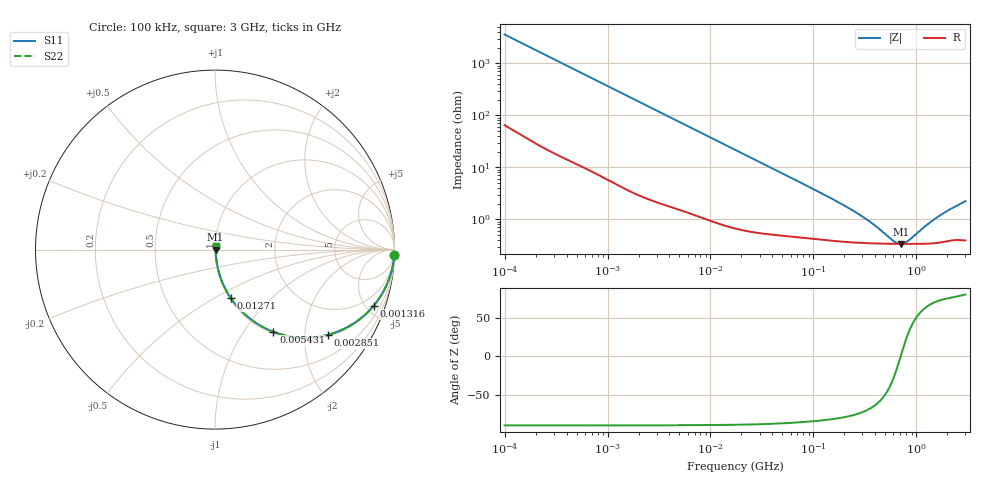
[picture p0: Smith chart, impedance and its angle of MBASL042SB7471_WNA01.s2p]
! MBASL042SB7471_WNA01  S-PARAMETER MODEL  ( Standard Model )
! Model Generated by TAIYO YUDEN Corporation (https://www.yuden.co.jp/en/)
! Version 1.0
! TAIYO YUDEN Control No. 250312
! Copyright(c) 2025 TAIYO YUDEN CO.,LTD. All Rights Reserved.
! Product Description (link to TY-COMPAS)
! https://ds.yuden.co.jp/TYCOMPAS/or/detail?pn=MBASL042SB7471KWNA01&u=M
! Products Name : Multilayer Ceramic Capacitors
! Characteristics :
!  Capacitance : 470 [pF] , Rated Voltage : 10 [V] , TCC : X7R
!  Case Size : 0.4 x 0.2 / 0.016 x 0.008 [mm/inch] , Thickness : 0.2 / 0.008 [mm/inch]
!  (Conditions: Temperature = 25 [degC] , DC Bias Voltage = 0 [V])
! External Node Assignments :
!  1  o---| |---o  2
! GND o---------o GND
! Frequency Range : 100kHz  -  3GHz  [ 401 STEP ]
# MHZ S RI R 50
! Freq[MHz].  S11 Real  S11 Imag  S21 Real  S21 Imag  S12 Real  S12 Imag  S22 Real  S22 Imag
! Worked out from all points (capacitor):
!   401 points, 100 kHz to 3 GHz, reference 50 ohm
!   read as one part in series: C = 440 pF near 105.3 kHz
!   lowest |Z| = 337 mohm at 708.5 MHz (marker M1)
!   series resonance near 704.3 MHz, so ESL is about 120 pH
!   S11 on the Smith chart (normalised r, x): 100 kHz: 2, -72; 1.316 MHz: 1.09, -5.62; 2.851 MHz: 1.04, -2.61; 5.431 MHz: 1.03, -1.38; 12.71 MHz: 1.02, -0.59; 3 GHz: 1.01, +0.04
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0.1  0.9987 -0.0277  0.00126 0.0277  0.00126 0.0277  0.9987 -0.0277
0.259498  0.9939 -0.0707  0.00613 0.0707  0.00613 0.0707  0.9939 -0.0707
0.562235  0.9748 -0.149  0.0252 0.149  0.0252 0.149  0.9748 -0.149
1.316074  0.884 -0.3126  0.116 0.3126  0.116 0.3126  0.884 -0.3126
1.937191  0.7822 -0.405  0.2178 0.405  0.2178 0.405  0.7822 -0.405
2.851441  0.628 -0.4749  0.372 0.4749  0.372 0.4749  0.628 -0.4749
3.161081  0.5799 -0.4849  0.4201 0.4849  0.4201 0.4849  0.5799 -0.4849
5.431059  0.3257 -0.4583  0.6743 0.4583  0.6743 0.4583  0.3257 -0.4583
8.202936  0.1796 -0.3723  0.8204 0.3723  0.8204 0.3723  0.1796 -0.3723
12.71297  0.0873 -0.2692  0.9127 0.2692  0.9127 0.2692  0.0873 -0.2692
17.7727  0.0492 -0.2013  0.9508 0.2013  0.9508 0.2013  0.0492 -0.2013
37.52708  0.0151 -0.0993  0.9849 0.0993  0.9849 0.0993  0.0151 -0.0993
97.38194  0.00572 -0.0386  0.9943 0.0386  0.9943 0.0386  0.00572 -0.0386
280.1453  0.00366 -0.0118  0.9963 0.0118  0.9963 0.0118  0.00366 -0.0118
391.6425  0.00348 -0.00692  0.9965 0.00692  0.9965 0.00692  0.00348 -0.00692
547.5153  0.00339 -0.00284  0.9966 0.00284  0.9966 0.00284  0.00339 -0.00284
639.0768  0.00337 -0.00109  0.9966 0.00109  0.9966 0.00109  0.00337 -0.00109
708.4746  0.00336 6.61e-05  0.9966 -6.61e-05  0.9966 -6.61e-05  0.00336 6.61e-05
826.9535  0.00336 0.00181  0.9966 -0.00181  0.9966 -0.00181  0.00336 0.00181
1249.01  0.00343 0.00681  0.9966 -0.00681  0.9966 -0.00681  0.00343 0.00681
1701.687  0.00369 0.0113  0.9963 -0.0113  0.9963 -0.0113  0.00369 0.0113
3000  0.00439 0.0218  0.9956 -0.0218  0.9956 -0.0218  0.00439 0.0218
